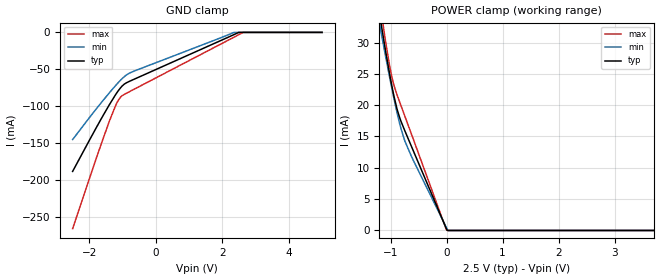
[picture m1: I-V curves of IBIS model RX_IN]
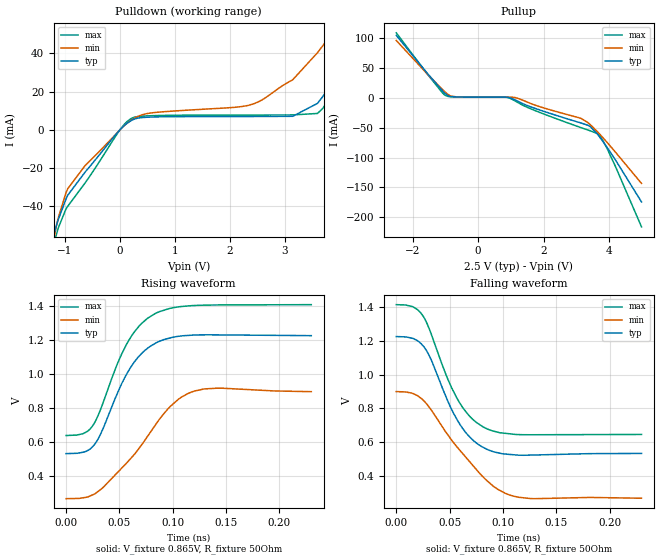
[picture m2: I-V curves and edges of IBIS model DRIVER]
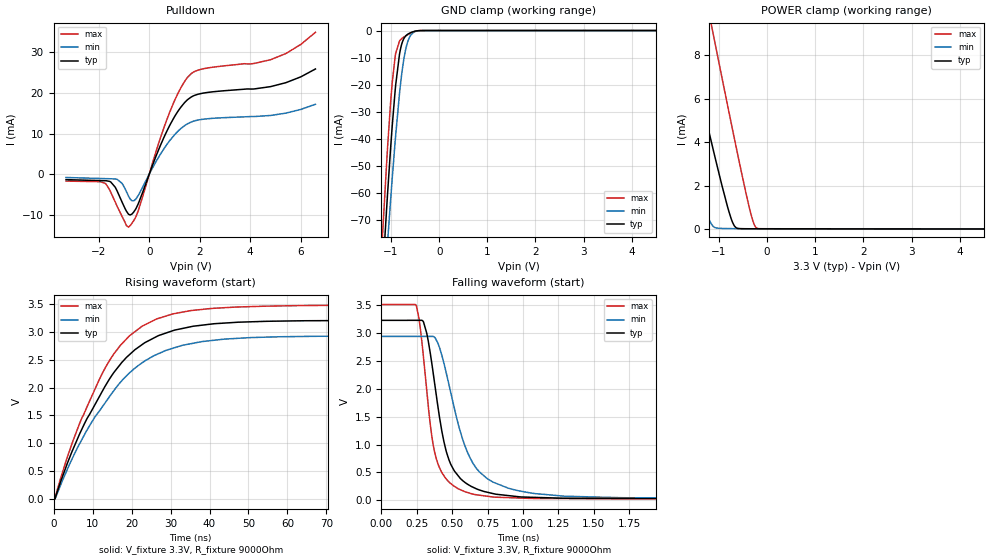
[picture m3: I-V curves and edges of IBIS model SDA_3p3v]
|Texas Instruments Incorporated
|2.5 Gbps/5.0 Gbps/8.0 Gbps 8 Channel PCI Express
|Repeater w/ Equalization & De-Emphasis
| Marketing part#   Voltage Range   Package-type   #pins
| DS80PCI800SQ   2.375to  3.6V   SQA54A   54
| DS80PCI800SQE   2.375to  3.6V   SQA54A   54
[IBIS Ver]   5.0
[File name]   ds80pci800.ibs
[File Rev]   1.0
[Date]   05/21/2012
[Source]   Texas Instruments Incorporated.
|   Analog-eLab, HPA
|   12500 TI Blvd
|   Dallas, TX -75243
|   For Support e-mail: elab_ibis@list.ti.com
[Notes]
 -Revision History:
 1.0: 4/12/2012
 - Initial version of the model
 - Initial Model generated from spice simulations
 - Models with trailing _3p3v are for 3.3V power supply operation and
   models with trailing _2p5v are for 2.5V power supply operation.
 - Non-monotonicity in combined Pulldown for SDA_3p3v reflects spice
   simulations and can be safely ignored.
 - c_comp although listed in numerical order of value are obtained from
   varying PVT conditions. IBIS model user is responsible for using appropriate
   c_comp to simulate for Signal Integrity.
[Disclaimer]
 This product is designed as an aid for customers of Texas Instruments.
 No warranties, either expressed or implied, with respect to this third
 party software (if any) or with respect to its fitness for any
 particular purpose is claimed by Texas Instruments or the author. The
 software (if any) is provided solely on an "as is" basis. The entire
 risk as to its quality and performance is with the customer
[Copyright] (C) Copyright 2012 Texas Instruments Incorporated.
   All rights reserved.
|   Component  DS80PCI800
[Component]   DS80PCI800
[Manufacturer]   Texas Instruments Incorporated
[Package] | 54pin SQA54A
|   typ   min   max
R_pkg   0   0   0
L_pkg   0   0   0
C_pkg   0   0   0
[Pin]   signal_name   model_name   R_pin   L_pin   C_pin
1   INB_0+   RX_IN
2   INB_0-   RX_IN
3   INB_1+   RX_IN
4   INB_1-   RX_IN
5   INB_2+   RX_IN
6   INB_2-   RX_IN
7   INB_3+   RX_IN
8   INB_3-   RX_IN
9   VDD   POWER
10   INA_0+   RX_IN
11   INA_0-   RX_IN
12   INA_1+   RX_IN
13   INA_1-   RX_IN
14   VDD   POWER
15   INA_2+   RX_IN
16   INA_2-   RX_IN
17   INA_3+   RX_IN
18   INA_3-   RX_IN
19   EQA1   IN_ML
20   EQA0   IN_ML
21   RATE   IN_ML
22   RXDET   IN_ML
23   RESERVED   NC
24   VIN   POWER
25   VDD_SEL   IN
26   SD_TH_READ_ENB   IN_ML
27   ALL_DONEB   OUT
28   OUTA_3-   DRIVER
29   OUTA_3+   DRIVER
30   OUTA_2-   DRIVER
31   OUTA_2+   DRIVER
32   OUTA_1-   DRIVER
33   OUTA_1+   DRIVER
34   OUTA_0-   DRIVER
35   OUTA_0+   DRIVER
36   VDD   POWER
37   OUTB_3-   DRIVER
38   OUTB_3+   DRIVER
39   OUTB_2-   DRIVER
40   OUTB_2+   DRIVER
41   VDD   POWER
42   OUTB_1-   DRIVER
43   OUTB_1+   DRIVER
44   OUTB_0-   DRIVER
45   OUTB_0+   DRIVER
46   EQB0/AD3   IN_ML
47   EQB1/AD2   IN_ML
48   ENSMB   IN
49   DEMA0_SDA   SDA
50   DEMA1_SCL   SDA
51   VDD   POWER
52   PRSNTB   IN
53   DEMB0_AD1   IN_ML
54   DEMB1_AD0   IN_ML
55   DAP   GND
[Package Model] llp54_ds80pci800
[Diff Pin]  inv_pin  vdiff  tdelay_typ tdelay_min tdelay_max
1   2   200mV   NA   NA   NA
3   4   200mV   NA   NA   NA
5   6   200mV   NA   NA   NA
7   8   200mV   NA   NA   NA
10   11   200mV   NA   NA   NA
12   13   200mV   NA   NA   NA
15   16   200mV   NA   NA   NA
17   18   200mV   NA   NA   NA
29   28   NA   NA   NA   NA
31   30   NA   NA   NA   NA
33   32   NA   NA   NA   NA
35   34   NA   NA   NA   NA
38   37   NA   NA   NA   NA
40   39   NA   NA   NA   NA
43   42   NA   NA   NA   NA
45   44   NA   NA   NA   NA
[Repeater Pin]
1  45
3  43
5  40
7  38
10 35
12 33
15 31
17 29
[Model Selector]   SDA
SDA_3p3v   SDA/SCL I/O with 3.3V operation
SDA_2p5v   SDA/SCL I/O with 2.5V operation
[Model Selector]   OUT
OUT_3p3v   Digital Output buffer with 3.3V operation
OUT_2p5v   Digital Output buffer with 2.5V operation
[Model Selector]   IN
IN_3p3v   Digital Input buffer with 3.3V operation
IN_2p5v   Digital Input buffer with 2.5V operation
[Model Selector]   IN_ML
IN_ML_3p3v   Digital Multilevel Input buffer with 3.3V operation
IN_ML_2p5v   Digital Multilevel Input buffer with 2.5V operation
|   Package model for DS80PCI800
[Define Package Model]  llp54_ds80pci800
[Manufacturer]  Texas Instruments,Inc.
[OEM]  Texas Instruments,Inc.
[Description]  Package Electrical model for LLP54-DS80PCI800
[Number Of Pins]  55
[Pin Numbers]
|Pin Num   Terminal Name
1   | LD1:1
2   | LD2:2
3   | LD3:3
4   | LD4:4
5   | LD5:5
6   | LD6:6
7   | LD7:7
8   | LD8:8
9   | LD9:9
10   | LD10:10
11   | LD11:11
12   | LD12:12
13   | LD13:13
14   | LD14:14
15   | LD15:15
16   | LD16:16
17   | LD17:17
18   | LD18:18
19   | LD19:19
20   | LD20:20
21   | LD21:21
22   | LD22:22
23   | LD23:23
24   | LD24:24
25   | LD25:25
26   | LD26:26
27   | LD27:27
28   | LD28:28
29   | LD29:29
30   | LD30:30
31   | LD31:31
32   | LD32:32
33   | LD33:33
34   | LD34:34
35   | LD35:35
36   | LD36:36
37   | LD37:37
38   | LD38:38
39   | LD39:39
40   | LD40:40
41   | LD41:41
42   | LD42:42
43   | LD43:43
44   | LD44:44
45   | LD45:45
46   | LD46:46
47   | LD47:47
48   | LD48:48
49   | LD49:49
50   | LD50:50
51   | LD51:51
52   | LD52:52
53   | LD53:53
54   | LD54:54
55   | LDAP:55
[Model Data]
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[End Model Data]
[End Package Model]
| Models and submodels in the file (10): RX_IN (Input), DRIVER (Output), SDA_3p3v (Open_drain), SDA_2p5v (Open_drain), OUT_3p3v (Output), OUT_2p5v (Output), IN_ML_3p3v (Input), IN_ML_2p5v (Input), IN_3p3v (Input), IN_2p5v (Input)
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[Model]   RX_IN
Model_type   Input
Vinl = 0.8
Vinh = 2
|   typ   min   max
C_comp   0.157pF   0.139pF   0.195pF
[Voltage Range]   2.5   2.375   2.625
[Temperature Range]   25   105   -40
[Power Clamp Reference]   2.5   2.375   2.625
[GND Clamp Reference]   0   -0   -0
[Algorithmic Model]
Executable Windows_VisualC++ExpressEdition9.0.30729_32 DS80PCI_Rx.dll DS80PCI_Rx.ami
Executable Linux_gcc4.6.1_64 DS80PCI_Rx_x64.so DS80PCI_Rx.ami
[End Algorithmic Model]
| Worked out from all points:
|   POWER clamp passes 1 mA (typ) near -0.04 V on its own axis
[GND Clamp]
|   Voltage   I(typ)   I(min)   I(max)
-2.5V     -188mA     -145mA     -265.5mA
-1.788V   -128.7mA   -103.3mA   -170.1mA
-1.383V   -96.79mA   -80.97mA   -118.4mA
-1.157V   -80.77mA   -69.3mA    -94.21mA
-1.052V   -74.5mA    -64.3mA    -87.18mA
-1.008V   -72.29mA   -62.31mA   -85.48mA
-880mV    -68.07mA   -57.46mA   -82.21mA
-625mV    -62.79mA   -51.83mA   -76.22mA
2.345V    -3.01mA    -123.6uA   -6.522mA
2.487V    -43.46uA   0A         -3.177mA
2.615V    0A         0A         -163.5uA
4.992V    0A         0A         0A
[POWER Clamp]
|   Voltage   I(typ)   I(min)   I(max)
-2.5V     113mA      101mA      126.7mA
-1.195V   34.45mA    32.91mA    36.67mA
-1.113V   29.93mA    28.92mA    31.58mA
-1.015V   24.9mA     24.38mA    26.22mA
-947.5mV  21.79mA    21.4mA     23.44mA
-880mV    19.25mA    18.64mA    21.55mA
-812.5mV  17.41mA    16.22mA    19.89mA
-745mV    15.92mA    14.28mA    18.25mA
-625mV    13.38mA    11.78mA    15.34mA
-62.5mV   1.532mA    1.553mA    1.568mA
12.5mV    56.91uA    193.5uA    0A
4.992V    0A         0A         0A
[Model]   DRIVER
Model_type   Output
Polarity   Non-Inverting
Vmeas = 0.865
Vref = 0.865
Cref = 1pF
Rref = 50
|   typ   min   max
C_comp   0.463pF   0.386pF   0.533pF
[Voltage Range]   2.5   2.375   2.625
[Temperature Range]   25   105   -40
[Pullup Reference]   2.5   2.375   2.625
[Pulldown Reference]   0   0   0
[Power Clamp Reference]   2.5   2.375   2.625
[GND Clamp Reference]   0   0   0
[Algorithmic Model]
Executable Windows_VisualC++ExpressEdition9.0.30729_32 DS80PCI_Tx.dll DS80PCI_Tx.ami
Executable Linux_gcc4.6.1_64 DS80PCI_Tx_x64.so DS80PCI_Tx.ami
[End Algorithmic Model]
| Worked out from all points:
|   slope of the pulldown table from 0 to 0.375 V, typ, clamps not added: 59 ohm
|   slope of the pullup table from 0 to 0.375 V, typ, clamps not added: 13.8 kohm
|   falling waveform, V_fixture 0.865V, R_fixture 50Ohm: 20-80 % time 30.6ps typ, 46.7ps min, 31.4ps max; typ from 1.23 V to 0.533 V
|   rising waveform, V_fixture 0.865V, R_fixture 50Ohm: 20-80 % time 31.9ps typ, 48.3ps min, 32.5ps max; typ from 0.533 V to 1.23 V
[Pulldown]
|   Voltage   I(typ)   I(min)   I(max)
-2.5V     -1.074A    -1.098A    -408.9mA
-1.3V     -65.37mA   -71.67mA   -72.59mA
-1.157V   -50.4mA    -50.83mA   -55.24mA
-947.5mV  -34.22mA   -30.83mA   -40mA
-625mV    -21.85mA   -18.47mA   -27.51mA
12.5mV    356.5uA    353.8uA    467.2uA
252.5mV   5.499mA    5.888mA    6.503mA
2.42V     6.991mA    13.52mA    7.738mA
3.14V     7.082mA    26.2mA     7.802mA
3.59V     13.86mA    40.36mA    8.578mA
3.688V    17.48mA    44.02mA    11.26mA
4.992V    73.4mA     95.56mA    71.14mA
[Pullup]
|   Voltage   I(typ)   I(min)   I(max)
-2.5V     104.9mA    96.36mA    109.2mA
-1.008V   7.433mA    9.92mA     4.453mA
-835mV    2.15mA     3.064mA    1.998mA
-625mV    1.52mA     1.453mA    1.529mA
912.5mV   936.5uA    1.242mA    618.9uA
1.16V     -4.181mA   182.1uA    -5.995mA
1.647V    -15.78mA   -10.25mA   -19.18mA
3.147V    -42.15mA   -34.48mA   -49.91mA
3.425V    -48.1mA    -44.75mA   -55.21mA
3.68V     -63.2mA    -58.69mA   -61.53mA
3.958V    -84.3mA    -75.62mA   -86.67mA
4.992V    -174.5mA   -143.4mA   -216.3mA
[Ramp]
R_load = 50
|   typ   min   max
dV/dt_r   0.415782/3.1895e-11   0.377209/4.80952e-11   0.461285/3.24209e-11
dV/dt_f   0.415782/3.05819e-11   0.379379/4.66388e-11   0.461707/3.13792e-11
[Falling Waveform]
V_fixture = 0.865V
V_fixture_min = 0.575V
V_fixture_max = 1.027V
R_fixture = 50Ohm
C_fixture = 0F
|   Time   V(typ)   V(min)   V(max)
0s        1.226V     899.5mV    1.415V
15.02ps   1.216V     889.6mV    1.404V
24.49ps   1.175V     853.3mV    1.353V
32.33ps   1.094V     794.7mV    1.249V
56.55ps   738.5mV    574.8mV    864.3mV
68.67ps   632.1mV    485mV      754.3mV
81.26ps   569.7mV    394.6mV    690.7mV
95.25ps   536.8mV    320.1mV    658.6mV
114.2ps   522.7mV    273.4mV    644.7mV
230ps     532.8mV    267.2mV    645.4mV
[Rising Waveform]
V_fixture = 0.865V
V_fixture_min = 0.575V
V_fixture_max = 1.027V
R_fixture = 50Ohm
C_fixture = 0F
|   Time   V(typ)   V(min)   V(max)
0s        532.8mV    268mV      639.1mV
15.81ps   540.8mV    273.2mV    649.8mV
24.49ps   570.9mV    289.4mV    692.3mV
31.91ps   641.5mV    319.5mV    785.2mV
56.55ps   997.1mV    476mV      1.173V
68.67ps   1.106V     565.7mV    1.283V
83.36ps   1.179V     697.4mV    1.355V
105.4ps   1.222V     852.1mV    1.395V
120.4ps   1.229V     900.4mV    1.403V
230ps     1.226V     896.7mV    1.408V
[Model]   SDA_3p3v
Model_type   Open_drain
Polarity   Non-Inverting
Vmeas = 1.65
Vref = 3.3
Cref = 1pF
Rref = 9000
|   typ   min   max
C_comp   0.949pF   0.893pF   1.043pF
[Voltage Range]   3.3   3   3.6
[Temperature Range]   25   105   -40
[Pullup Reference]   3.3   3   3.6
[Pulldown Reference]   0   0   -0
[Power Clamp Reference]   3.3   3   3.6
[GND Clamp Reference]   0   -0   0
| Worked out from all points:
|   slope of the pulldown table from 0 to 0.495 V, typ, clamps not added: 63.4 ohm
|   GND clamp passes 1 mA (typ) near -0.62 V on its own axis
|   POWER clamp passes 1 mA (typ) near -0.82 V on its own axis
|   falling waveform, V_fixture 3.3V, R_fixture 9000Ohm: 20-80 % time 139ps typ, 210ps min, 104ps max; typ from 3.23 V to 0.021 V
|   rising waveform, V_fixture 3.3V, R_fixture 9000Ohm: 20-80 % time 15.6ns typ, 16.9ns min, 14.3ns max; typ from 0.021 V to 3.21 V
[Pulldown]
|   Voltage   I(typ)   I(min)   I(max)
-3.3V     -1.332mA   -798uA     -1.685mA
-1.756V   -1.589mA   -1.077mA   -2.211mA
-1.528V   -1.894mA   -1.115mA   -4.392mA
-1.27V    -4.151mA   -1.258mA   -7.916mA
-815.1mV  -9.859mA   -5.451mA   -12.98mA
-528mV    -8.462mA   -6.067mA   -10.42mA
699.6mV   10.6mA     7.313mA    13.44mA
1.115V    15.26mA    10.42mA    19.59mA
1.531V    18.39mA    12.45mA    23.9mA
2.165V    19.97mA    13.54mA    25.95mA
4.818V    21.55mA    14.45mA    28.17mA
6.59V     25.87mA    17.2mA     34.89mA
[GND Clamp]
|   Voltage   I(typ)   I(min)   I(max)
-3.3V     -766.2mA   -698.7mA   -829.3mA
-1.191V   -94.73mA   -109.2mA   -79.98mA
-1.082V   -63.02mA   -80.79mA   -45.97mA
-1.073V   -60.27mA   -78.28mA   -43.13mA
-1.013V   -44.43mA   -63.54mA   -27.47mA
-973.5mV  -34.71mA   -54.11mA   -18.79mA
-904.2mV  -20.11mA   -38.66mA   -8.438mA
-825mV    -8.775mA   -23.36mA   -3.898mA
-716.1mV  -2.466mA   -8.7mA     -2.193mA
-587.4mV  -757.9uA   -1.633mA   -914.3uA
-270.6mV  -1.2uA     -2.7uA     -794.8nA
6.59V     0A         0A         0A
[POWER Clamp]
|   Voltage   I(typ)   I(min)   I(max)
-3.3V     25.04mA    17.6mA     33.7mA
-2.33V    15.39mA    9.309mA    22.61mA
-1.805V   10.23mA    4.926mA    16.66mA
-1.597V   8.207mA    3.241mA    14.32mA
-1.32V    5.54mA     1.139mA    11.21mA
-1.132V   3.765mA    145.8uA    9.115mA
-1.092V   3.397mA    73.28uA    8.676mA
-825mV    1.044mA    18.61uA    5.736mA
-686.4mV  162uA      14.01uA    4.234mA
-359.7mV  9.294uA    7.715uA    893.2uA
-211.2mV  8.711uA    7.131uA    34.86uA
6.59V     0A         0A         0A
[Ramp]
R_load = 9000
|   typ   min   max
dV/dt_r   1.91256/1.5556e-08   1.73921/1.68669e-08   2.08187/1.43224e-08
dV/dt_f   1.92377/1.39153e-10   1.74696/2.09717e-10   2.09556/1.04188e-10
[Falling Waveform]
V_fixture = 3.3V
V_fixture_min = 3V
V_fixture_max = 3.6V
R_fixture = 9000Ohm
C_fixture = 0F
|   Time   V(typ)   V(min)   V(max)
0s        3.227V     2.939V     3.511V
247.4ps   3.228V     2.94V      3.484V
297ps     3.201V     2.94V      2.57V
365ps     2.296V     2.939V     1.004V
454ps     919.5mV    2.327V     394.8mV
573.4ps   355.4mV    1.099V     173.5mV
666ps     212.9mV    590.1mV    102mV
791.1ps   119.9mV    324.7mV    58.75mV
1.052ns   55.76mV    133.8mV    35.02mV
100ns     21.15mV    27.42mV    18.47mV
[Rising Waveform]
V_fixture = 3.3V
V_fixture_min = 3V
V_fixture_max = 3.6V
R_fixture = 9000Ohm
C_fixture = 0F
|   Time   V(typ)   V(min)   V(max)
0s        21.15mV    27.43mV    18.5mV
426.2ps   21.45mV    10.89mV    33.93mV
3.581ns   648.8mV    540.5mV    763mV
6.726ns   1.175V     998.2mV    1.364V
13.59ns   2.066V     1.762V     2.394V
19.5ns    2.591V     2.264V     2.928V
26.45ns   2.914V     2.593V     3.23V
33.05ns   3.059V     2.757V     3.352V
43.84ns   3.155V     2.868V     3.431V
100ns     3.209V     2.926V     3.488V
